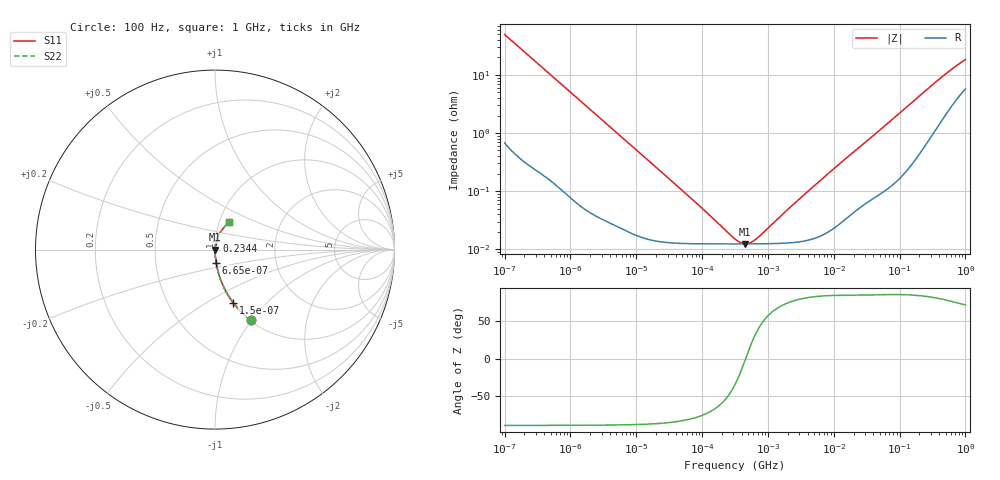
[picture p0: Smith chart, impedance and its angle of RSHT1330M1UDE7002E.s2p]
! RSHT1330M1UDE7002E  S-PARAMETER MODEL  (General Type)
! Model Generated by ELNA Corporation (http://www.ty-top.com)
! Version 1.0
! ELNA Control No.240229
! Copyright (c) 2024 ELNA CO.,LTD. All Rights Reserved.
! Products Name : CONDUCTIVE POLYMER HYBRID ALUMINUM ELECTROLYTIC CAPACITORS
! Characteristics :
!  Capacitance  :  33uF  ,  Rated voltage  :  50V
!  Operating Temp. Range  :  -55 to +105 degC  ,  Endurance  :  10000hr at 105 degC
!  Dimension D  :  6.3mm  ,  Dimension L  :  7.7mm
! Frequency Range : 100Hz - 1GHz
! External Node Assignments :
!  1  o---| |---o  2
# MHz S RI R 50
!Freq[MHz].  S11 Real  S11 Imag  S21 Real  S21 Imag  S12 Real  S12 Imag  S22 Real  S22 Imag
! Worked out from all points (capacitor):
!   401 points, 100 Hz to 1 GHz, reference 50 ohm
!   read as one part in series: C = 32.1 uF near 108 Hz
!   lowest |Z| = 12.4 mohm at 454.5 kHz (marker M1)
!   series resonance near 458.2 kHz, so ESL is about 3.8 nH
!   S11 on the Smith chart (normalised r, x): 100 Hz: 1.01, -0.99; 150 Hz: 1.01, -0.66; 665 Hz: 1.00, -0.15; 234.4 MHz: 1.01, +0.10; 1 GHz: 1.11, +0.35
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0.0001  0.2005 -0.3936  0.7995 0.3936  0.7995 0.3936  0.2005 -0.3936
0.00015  0.102 -0.2965  0.898 0.2965  0.898 0.2965  0.102 -0.2965
0.000198  0.0616 -0.2342  0.9384 0.2342  0.9384 0.2342  0.0616 -0.2342
0.000309  0.0274 -0.1564  0.9726 0.1564  0.9726 0.1564  0.0274 -0.1564
0.000665  0.0068 -0.0749  0.9932 0.0749  0.9932 0.0749  0.0068 -0.0749
0.001488  0.00168 -0.0339  0.9983 0.0339  0.9983 0.0339  0.00168 -0.0339
0.004241  0.000416 -0.012  0.9996 0.012  0.9996 0.012  0.000416 -0.012
0.022131  0.000141 -0.00232  0.9999 0.00232  0.9999 0.00232  0.000141 -0.00232
0.090678  0.000124 -0.000546  0.9999 0.000546  0.9999 0.000546  0.000124 -0.000546
0.316228  0.000123 -8.54e-05  0.9999 8.54e-05  0.9999 8.54e-05  0.000123 -8.54e-05
0.386812  0.000123 -3.83e-05  0.9999 3.83e-05  0.9999 3.83e-05  0.000123 -3.83e-05
0.454465  0.000124 -1.82e-06  0.9999 1.82e-06  0.9999 1.82e-06  0.000124 -1.82e-06
0.555904  0.000124 4.38e-05  0.9999 -4.38e-05  0.9999 -4.38e-05  0.000124 4.38e-05
0.679986  0.000124 9.12e-05  0.9999 -9.12e-05  0.9999 -9.12e-05  0.000124 9.12e-05
1.938653  0.000128 0.000449  0.9999 -0.000449  0.9999 -0.000449  0.000128 0.000449
4.704354  0.000151 0.00114  0.9998 -0.00114  0.9998 -0.00114  0.000151 0.00114
12.37371  0.000282 0.00296  0.9997 -0.00296  0.9997 -0.00296  0.000282 0.00296
69.9842  0.00139 0.0154  0.9986 -0.0154  0.9986 -0.0154  0.00139 0.0154
234.4229  0.00807 0.0497  0.9919 -0.0497  0.9919 -0.0497  0.00807 0.0497
546.3866  0.0343 0.1034  0.9657 -0.1034  0.9657 -0.1034  0.0343 0.1034
817.523  0.0617 0.1358  0.9383 -0.1358  0.9383 -0.1358  0.0617 0.1358
1000  0.0791 0.152  0.9209 -0.152  0.9209 -0.152  0.0791 0.152
